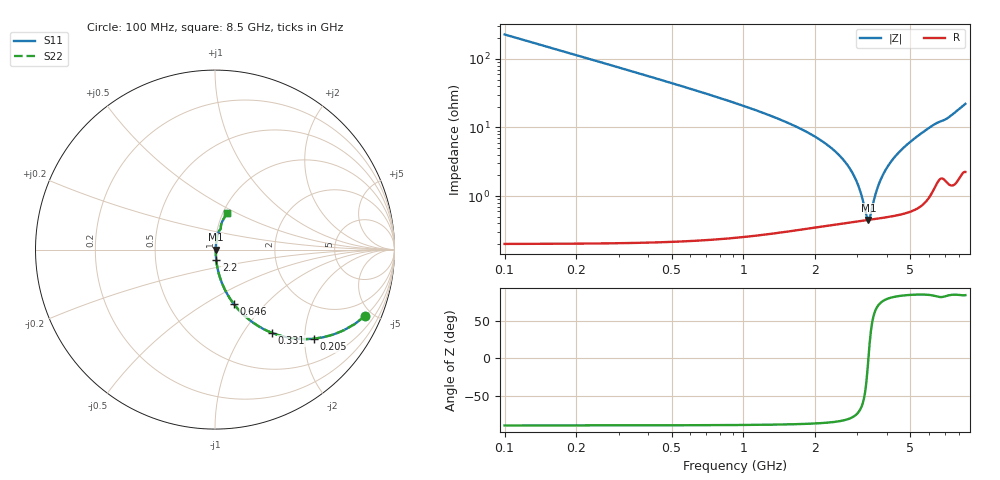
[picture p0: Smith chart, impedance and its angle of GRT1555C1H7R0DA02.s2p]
!Murata Part Number: GRT1555C1H7R0DA02
!These Parameters are Measured in Series Mode Connection
!Data Generated on Jun 19, 2026
!  o--ll--o
!Port1  Port2
!  o------o
!Operation Temp=25[degC], DC Bias Voltage=0[V]
!Freq. Start=100[MHz] Stop=9[GHz] 401[Steps]
# Hz S RI R 50
!Freq.(Hz) S11(Real) S11(Imag) S21(Real) S21(Imag) S12(Real) S12(Imag) S22(Real) S22(Imag)
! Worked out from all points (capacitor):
!   401 points, 100 MHz to 8.5 GHz, reference 50 ohm
!   read as one part in series: C = 7 pF near 142 MHz
!   lowest |Z| = 449 mohm at 3.334 GHz (marker M1)
!   series resonance near 3.337 GHz, so ESL is about 320 pH
!   S11 on the Smith chart (normalised r, x): 100 MHz: 1.00, -4.54; 205 MHz: 1.00, -2.21; 331 MHz: 1.00, -1.36; 646 MHz: 1.00, -0.68; 2.2 GHz: 1.01, -0.12; 8.5 GHz: 1.04, +0.44
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1e8  0.8374 -0.3685  0.1626 0.3685  0.1626 0.3685  0.8374 -0.3685
2.05e8  0.5496 -0.4966  0.4504 0.4966  0.4504 0.4966  0.5496 -0.4966
3.31e8  0.3168 -0.4637  0.6832 0.4637  0.6832 0.4637  0.3168 -0.4637
4.57e8  0.1935 -0.3928  0.8065 0.3928  0.8065 0.3928  0.1935 -0.3928
6.46e8  0.1045 -0.3026  0.8955 0.3026  0.8955 0.3026  0.1045 -0.3026
1.003e9  0.043 -0.1968  0.957 0.1968  0.957 0.1968  0.043 -0.1968
1.507e9  0.0171 -0.1177  0.9829 0.1177  0.9829 0.1177  0.0171 -0.1177
2.2e9  0.00704 -0.0581  0.993 0.0581  0.993 0.0581  0.00704 -0.0581
2.62e9  0.00509 -0.0333  0.9949 0.0333  0.9949 0.0333  0.00509 -0.0333
2.914e9  0.00453 -0.0187  0.9955 0.0187  0.9955 0.0187  0.00453 -0.0187
3.061e9  0.00443 -0.0119  0.9956 0.0119  0.9956 0.0119  0.00443 -0.0119
3.271e9  0.00443 -0.00278  0.9956 0.00278  0.9956 0.00278  0.00443 -0.00278
3.334e9  0.00446 -0.000144  0.9955 0.000144  0.9955 0.000144  0.00446 -0.000144
3.397e9  0.00451 0.00245  0.9955 -0.00245  0.9955 -0.00245  0.00451 0.00245
3.607e9  0.00476 0.0108  0.9952 -0.0108  0.9952 -0.0108  0.00476 0.0108
3.754e9  0.00501 0.0165  0.995 -0.0165  0.995 -0.0165  0.00501 0.0165
3.985e9  0.00553 0.0251  0.9945 -0.0251  0.9945 -0.0251  0.00553 0.0251
4.3e9  0.00646 0.0364  0.9935 -0.0364  0.9935 -0.0364  0.00646 0.0364
4.888e9  0.00898 0.0568  0.991 -0.0568  0.991 -0.0568  0.00898 0.0568
5.707e9  0.0152 0.0855  0.9848 -0.0855  0.9848 -0.0855  0.0152 0.0855
7.114e9  0.0324 0.1279  0.9676 -0.1279  0.9676 -0.1279  0.0324 0.1279
8.5e9  0.0653 0.2013  0.9347 -0.2013  0.9347 -0.2013  0.0653 0.2013
